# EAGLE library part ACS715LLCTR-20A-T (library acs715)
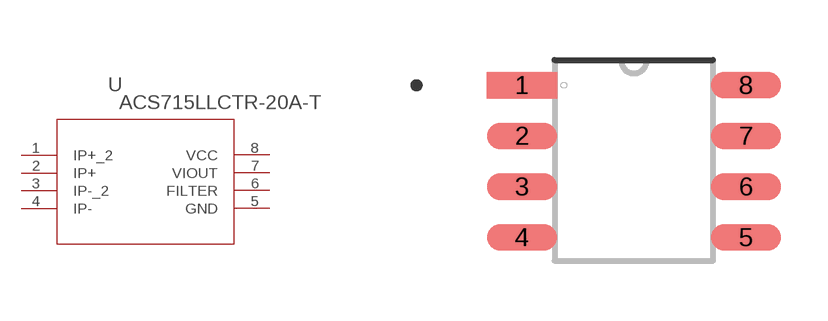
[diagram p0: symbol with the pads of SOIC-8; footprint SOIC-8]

Designator prefix U

## ACS715LLCTR-20A-T (MANUFACTURER_PART_NUMBER: ACS715LLCTR20AT; VENDOR: Allegro Microsystems Inc.)  [SOIC-8]
1  IP+_2  in
2  IP+  in
3  IP-_2  out
4  IP-  out
5  GND  pwr
6  FILTER  pas
7  VIOUT  out
8  VCC  pwr

## Footprint SOIC-8 (pad centres in mm)
smd 1.753 x 0.66: 1 -2.8,1.905; 2 -2.8,0.635; 3 -2.8,-0.635; 4 -2.8,-1.905; 5 2.8,-1.905; 6 2.8,-0.635; 7 2.8,0.635; 8 2.8,1.905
